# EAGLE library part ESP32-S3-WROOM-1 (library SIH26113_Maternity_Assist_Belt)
Espressif ESP32-S3-WROOM-1-N8R2. Xtensa LX7 dual-core, Wi-Fi b/g/n + Bluetooth LE 5, 8 MB flash, 2 MB quad-SPI PSRAM, PCB antenna. Pin map from datasheet v1.8 Table 3-1. IO35/36/37 are free on the -N8R2 (quad PSRAM) variant only.
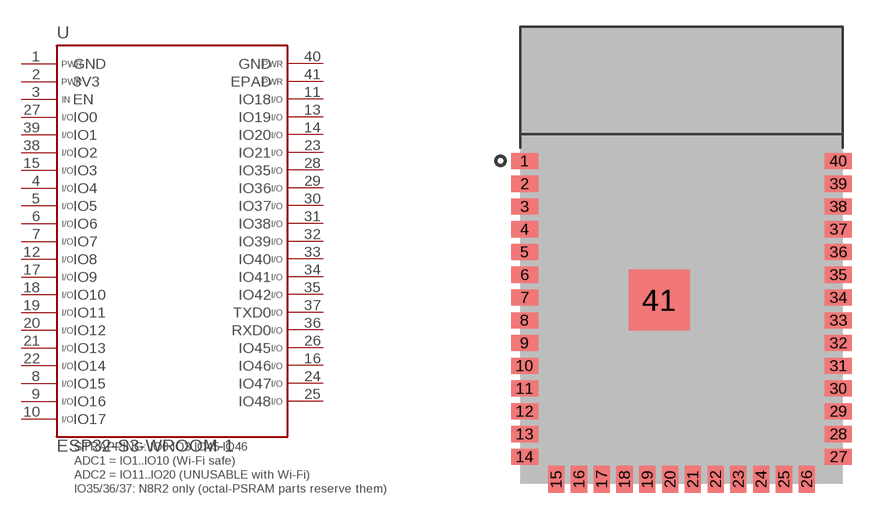
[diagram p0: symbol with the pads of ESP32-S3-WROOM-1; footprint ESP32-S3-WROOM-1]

Designator prefix U

## ESP32-S3-WROOM-1  [ESP32-S3-WROOM-1]
1  GND  pwr
2  3V3  pwr
3  EN  in
4  IO4
5  IO5
6  IO6
7  IO7
8  IO15
9  IO16
10  IO17
11  IO18
12  IO8
13  IO19
14  IO20
15  IO3
16  IO46
17  IO9
18  IO10
19  IO11
20  IO12
21  IO13
22  IO14
23  IO21
24  IO47
25  IO48
26  IO45
27  IO0
28  IO35
29  IO36
30  IO37
31  IO38
32  IO39
33  IO40
34  IO41
35  IO42
36  RXD0
37  TXD0
38  IO2
39  IO1
40  GND  pwr
41  EPAD  pwr

## Footprint ESP32-S3-WROOM-1 (pad centres in mm)
Espressif ESP32-S3-WROOM-1 module land pattern. Source: ESP32-S3-WROOM-1/1U datasheet v1.8 Fig.11-1 + Fig.10-1. 40 lands 1.5x0.9 mm, 1.27 mm pitch, 17.5 mm row spacing, pin 1 at 7.49 mm from the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
smd 1.5 x 0.9: 1 -8.75,5.26; 2 -8.75,3.99; 3 -8.75,2.72; 4 -8.75,1.45; 5 -8.75,0.18; 6 -8.75,-1.09; 7 -8.75,-2.36; 8 -8.75,-3.63; 9 -8.75,-4.9; 10 -8.75,-6.17; 11 -8.75,-7.44; 12 -8.75,-8.71; 13 -8.75,-9.98; 14 -8.75,-11.25; 27 8.75,-11.25; 28 8.75,-9.98; 29 8.75,-8.71; 30 8.75,-7.44; 31 8.75,-6.17; 32 8.75,-4.9; 33 8.75,-3.63; 34 8.75,-2.36; 35 8.75,-1.09; 36 8.75,0.18; 37 8.75,1.45; 38 8.75,2.72; 39 8.75,3.99; 40 8.75,5.26
smd 0.9 x 1.5: 15 -6.985,-12.5; 16 -5.715,-12.5; 17 -4.445,-12.5; 18 -3.175,-12.5; 19 -1.905,-12.5; 20 -0.635,-12.5; 21 0.635,-12.5; 22 1.905,-12.5; 23 3.175,-12.5; 24 4.445,-12.5; 25 5.715,-12.5; 26 6.985,-12.5
smd 3.4 x 3.4: 41 -1.25,-2.5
